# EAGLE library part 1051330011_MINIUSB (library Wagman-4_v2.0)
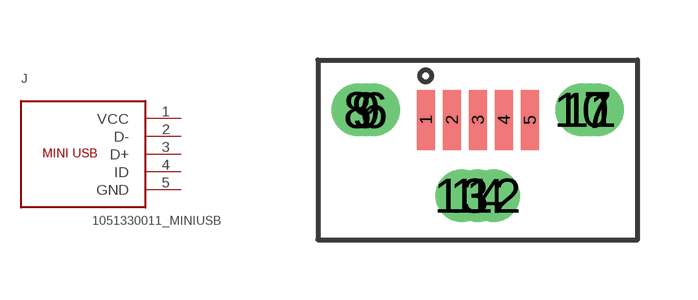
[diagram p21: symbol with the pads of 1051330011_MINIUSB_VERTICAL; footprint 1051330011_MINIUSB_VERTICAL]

Designator prefix J

## 1051330011_MINIUSB  [1051330011_MINIUSB_VERTICAL]
1  VCC  pas
2  D-  pas
3  D+  pas
4  ID  pas
5  GND  pas
6  6  pas
7  7  pas
8  6  pas
9  6  pas
10  7  pas
11  7  pas
12  12  pas
13  12  pas
14  12  pas

## Footprint 1051330011_MINIUSB_VERTICAL (pad centres in mm)
smd 0.45 x 1.5: 1 -1.3,0; 2 -0.65,0; 3 0,0; 4 0.65,0; 5 1.3,0
drill 0.8: 6 -2.6,0.25; 7 3,0.25; 8 -3,0.25; 9 -2.8,0.25; 10 2.6,0.25; 11 2.8,0.25; 12 0.4,-1.9; 13 -0.4,-1.9; 14 0,-1.9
